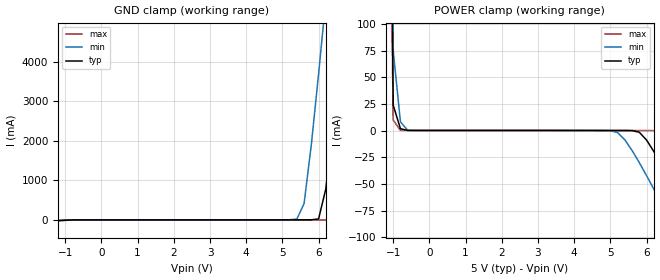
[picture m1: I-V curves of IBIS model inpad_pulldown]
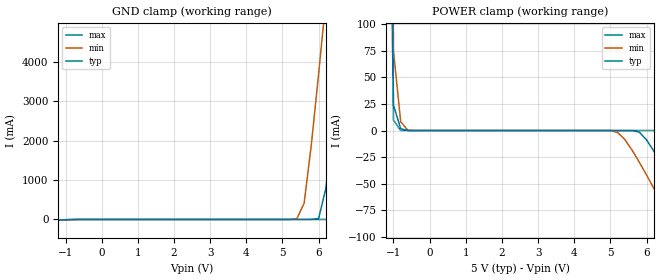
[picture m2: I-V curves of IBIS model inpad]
[IBIS Ver]   2.1
[File Name]   dac904e5.ibs
[File Rev]   1.1
[Source]   Preliminary IBIS Model Generated Manually
[Notes]
   Package information estimated
[Disclaimer]   This information is for modeling purposes only
[Copyright]   (c) 2004, Texas Instruments Inc.
[Component]   tssop28
[Manufacturer]   Texas Instruments
[Package]
| Variable   Typ   Min   Max
R_pkg   0.1   0.1   0.1
L_pkg   3.0nH   3.0nH   3.0nH
C_pkg   3.0pF   3.0pF   3.0pF
[Pin]   signal_name   model_name   R_pin  L_pin   C_pin
   1   bit1   inpad   0.1   3.0nH   3.0pF
   2   bit2   inpad   0.1   3.0nH   3.0pF
   3   bit3   inpad   0.1   3.0nH   3.0pF
   4   bit4   inpad   0.1   3.0nH   3.0pF
   5   bit5   inpad   0.1   3.0nH   3.0pF
   6   bit6   inpad   0.1   3.0nH   3.0pF
   7   bit7   inpad   0.1   3.0nH   3.0pF
   8   bit8   inpad   0.1   3.0nH   3.0pF
   9   bit9   inpad   0.1   3.0nH   3.0pF
   10   bit10   inpad   0.1   3.0nH   3.0pF
   11   bit11   inpad   0.1   3.0nH   3.0pF
   12   bit12   inpad   0.1   3.0nH   3.0pF
|  13   bit13   inpad   0.1   3.0nH   3.0pF
|  14   bit14   inpad   0.1   3.0nH   3.0pF
   15   pd   inpad_pulldown   0.1   3.0nH   3.0pF
   16   int_ext_n   inpad   0.1   3.0nH   3.0pF
|  17   refin   0.1   3.0nH   3.0pF
|  18   fsa   0.1   3.0nH   3.0pF
|  19   bw   0.1   3.0nH   3.0pF
   20   agnd   GND   0.1   3.0nH   3.0pF
|  21   ioutb   0.1   3.0nH   3.0pF
|  22   iout   0.1   3.0nH   3.0pF
|  23   byp   0.1   3.0nH   3.0pF
   24   va   POWER   0.1   3.0nH   3.0pF
|  25   nc   0.1   3.0nH   3.0pF
   26   dgnd   GND   0.1   3.0nH   3.0pF
   27   vd   POWER   0.1   3.0nH   3.0pF
   28   clk   inpad   0.1   3.0nH   3.0pF
| End of package information
| Models and submodels in the file (2): inpad_pulldown (Input), inpad (Input)
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|   Model inpad_pulldown
[Model]   inpad_pulldown
Model_type   Input
Polarity   Non-Inverting
| signals   A, Y
Vinl = 1.2V
Vinh = 3.5V
|   typ   min   max
C_comp   1.5p   1.5p   1.5p
|   typ   min   max
[Temperature Range]   25   -40.0   100
|   typ   min   max
[Voltage Range]   5.00V   4.50V   5.50V
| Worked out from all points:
|   GND clamp passes 1 mA (typ) near -0.72 V on its own axis
|   POWER clamp passes 1 mA (typ) near -0.71 V on its own axis
[GND_clamp]
|   Voltage   I(typ)   I(min)   I(max)
-5V       -276.9mA   -278.6mA   -279mA
-1V       -8.91mA    -13.47mA   -5.081mA
5.4V      68.42uA    19.54mA    132.5uA
5.6V      70.09uA    413mA      132.6uA
5.8V      1.718mA    1.905A     132.6uA
6V        23.55mA    3.69A      132.7uA
6.2V      781.5mA    5.558A     132.9uA
6.6V      4.333A     9.39A      57.25mA
6.8V      6.239A     11.33A     1.351A
7V        8.169A     13.28A     3.178A
7.2V      10.12A     15.23A     5.084A
10V       37.77A     42.9A      32.71A
[POWER_clamp]
|   Voltage   I(typ)   I(min)   I(max)
-5V       37.77A     37.94A     37.68A
-1.2V     785.5mA    1.091A     539.7mA
-1V       23.8mA     74.85mA    9.767mA
-800mV    1.719mA    8.14mA     165.2uA
-600mV    70.23uA    227.8uA    132.7uA
5.2V      -8.065uA   -1.868mA   19.3uA
5.8V      -1.599mA   -30.08mA   -20.48uA
6.4V      -31.45mA   -67.69mA   -1.617mA
6.8V      -56.93mA   -93.98mA   -21.47mA
7.4V      -96.89mA   -134.3mA   -60.57mA
8V        -137.8mA   -175.1mA   -101.8mA
10V       -276.9mA   -313.4mA   -243.2mA
|   Model inpad
[Model]   inpad
Model_type   Input
Polarity   Non-Inverting
| signals   A, Y
Vinl = 1.2V
Vinh = 3.5V
|   typ   min   max
C_comp   1.5p   1.5p   1.5p
|   typ   min   max
[Temperature Range]   25   -40.0   100
|   typ   min   max
[Voltage Range]   5.00V   4.50V   5.50V
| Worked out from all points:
|   GND clamp passes 1 mA (typ) near -0.73 V on its own axis
|   POWER clamp passes 1 mA (typ) near -0.72 V on its own axis
[GND_clamp]
|   Voltage   I(typ)   I(min)   I(max)
-5V       -275.1mA   -277.3mA   -275.7mA
-1V       -8.742mA   -13.28mA   -4.917mA
5.4V      3.308nA    19.53mA    1.734nA
5.6V      1.955uA    413mA      1.833nA
5.8V      1.689mA    1.905A     1.978nA
6V        23.54mA    3.69A      2.252nA
6.2V      781.5mA    5.558A     275.8nA
6.6V      4.333A     9.39A      57.23mA
6.8V      6.239A     11.33A     1.351A
7V        8.169A     13.28A     3.178A
7.2V      10.12A     15.23A     5.084A
10V       37.77A     42.9A      32.71A
[POWER_clamp]
|   Voltage   I(typ)   I(min)   I(max)
-5V       37.77A     37.94A     37.68A
-1.2V     785.5mA    1.091A     539.7mA
-1V       23.79mA    74.84mA    9.733mA
-800mV    1.69mA     8.132mA    39.32uA
-600mV    2.115uA    204uA      2.765nA
5.2V      -2.615nA   -1.794mA   -1.928nA
5.8V      -1.532mA   -29.79mA   -2.476nA
6.4V      -31.1mA    -67.22mA   -1.535mA
6.8V      -56.41mA   -93.39mA   -21.04mA
7.4V      -96.11mA   -133.5mA   -59.65mA
8V        -136.8mA   -174.2mA   -100.4mA
10V       -275.1mA   -311.9mA   -240.3mA
